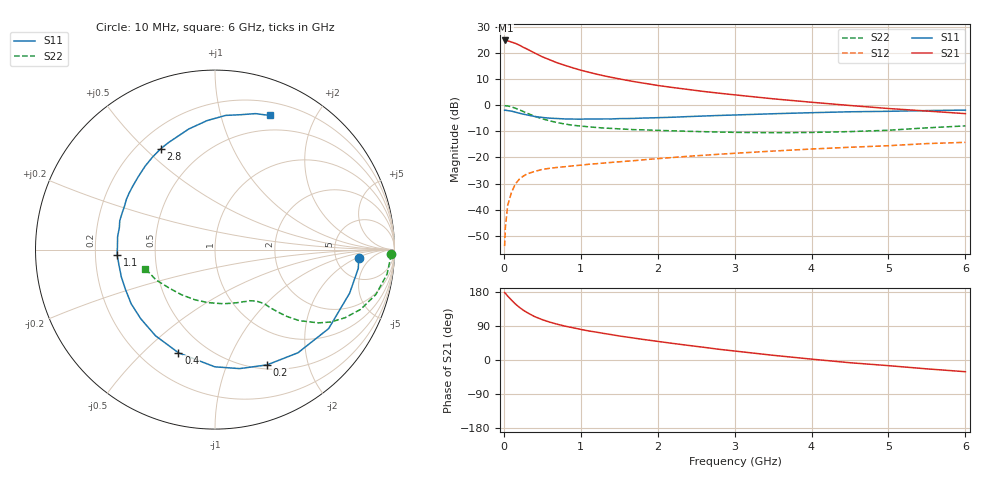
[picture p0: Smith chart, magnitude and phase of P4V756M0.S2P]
! SIEMENS Small Signal Semiconductors
! BFP182
! Si NPN RF Bipolar Junction Transistor in SOT143
! VCE = 0.75 V  IC = 6 mA
! Common Emitter S-Parameters:  March  1996
# GHz  S  MA  R  50
!  f  S11  S21  S12  S22
! GHz  MAG  ANG  MAG  ANG  MAG  ANG  MAG  ANG
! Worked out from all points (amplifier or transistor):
!   36 points, 10 MHz to 6 GHz, reference 50 ohm
!   highest |S21| = 24.8 dB at 20 MHz (marker M1)
!   |S21| within 3 dB of that: start of sweep to 280.5 MHz
!   unconditionally stable (mu >= 1): 1.275 GHz to end of sweep
!   at 250 MHz: K = 0.26, MSG = 24.7 dB, |S12| = -27.2 dB
!   at 1.4 GHz: K = 1.06, MAG = 14.8 dB, |S12| = -21.9 dB
!   at 6 GHz: K = 1.06, MAG = 4.0 dB, |S12| = -14.2 dB
!   S11 on the Smith chart (normalised r, x): 10 MHz: 8.42, -2.30; 200 MHz: 0.55, -1.40; 400 MHz: 0.35, -0.65; 1.1 GHz: 0.29, -0.03; 2.8 GHz: 0.29, +0.56; 6 GHz: 0.33, +1.44
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0.01  0.8012 -3.5  17.14 178.0  0.002 79.1  0.9808 -1.5
0.02  0.8053 -7.4  17.41 175.9  0.0046 85.6  0.9778 -3.2
0.05  0.7885 -17.9  17.18 168.7  0.0121 83.8  0.9685 -8.1
0.1  0.7711 -34.8  16.23 158.0  0.0216 70.8  0.9306 -15.6
0.15  0.7376 -51.2  15.35 147.9  0.0311 63.9  0.8773 -22.3
0.2  0.7047 -65.7  14.21 139.3  0.0382 58.6  0.8185 -27.6
0.25  0.6771 -78.3  12.95 131.8  0.0436 53.3  0.7613 -32.0
0.3  0.6531 -90.1  11.95 125.5  0.0483 48.8  0.7064 -35.3
0.4  0.6099 -109.5  10.03 114.5  0.054 42.9  0.6148 -40.1
0.5  0.5834 -124.6  8.472 106.4  0.0591 38.7  0.5495 -42.8
0.6  0.5653 -137.0  7.39 99.8  0.0621 36.4  0.5011 -44.5
0.7  0.5562 -147.1  6.444 94.1  0.0646 34.9  0.4636 -45.8
0.9  0.5436 -163.7  5.193 85.0  0.0692 33.3  0.4141 -47.4
1.1  0.546 -176.8  4.31 76.8  0.0739 32.5  0.3864 -49.4
1.3  0.5474 172.4  3.665 70.1  0.0782 32.1  0.3665 -51.5
1.6  0.5561 158.4  3.003 60.5  0.0849 32.5  0.3467 -55.3
2.2  0.5899 136.4  2.182 43.7  0.1 31.7  0.3238 -65.4
2.8  0.6378 118.4  1.7 28.2  0.1153 29.2  0.3068 -78.5
3.5  0.6875 102.3  1.329 12.4  0.1326 25.4  0.298 -97.4
4.5  0.7499 85.5  0.989 -7.2  0.1569 19.2  0.3129 -126.4
5.5  0.7906 73.4  0.774 -23.4  0.1844 12.8  0.3692 -152.7
6  0.8072 67.8  0.691 -30.9  0.1948 8.2  0.4021 -164.5
